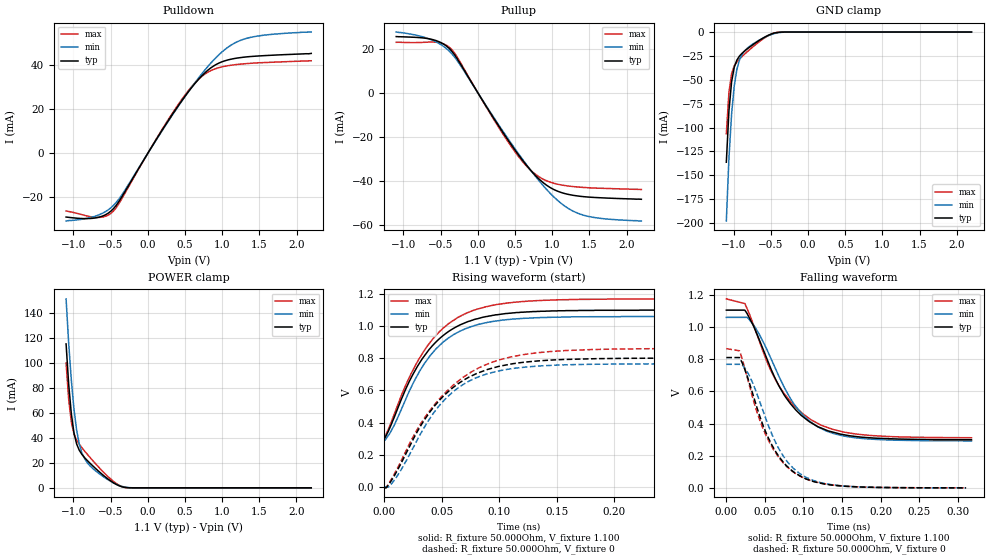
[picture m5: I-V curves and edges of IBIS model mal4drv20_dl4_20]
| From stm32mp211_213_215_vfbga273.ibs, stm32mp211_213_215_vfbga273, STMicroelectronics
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[Model] mal4drv20_dl4_20
Model_type   I/O
Polarity   Non-Inverting
Enable   Active-High
C_comp   1.837pF   1.837pF   1.849pF
C_comp_pullup   942.491fF   934.703fF   950.576fF
C_comp_pulldown 782.742fF   781.933fF   799.826fF
Vinh = 453.000mV
Vinl = 333.000mV
Vmeas = 393.000mV
Vref = 0.00V
Rref = 50Ohms
Cref = 0pF
[Model Spec]
Vinh   453.000mV   439.000mV   478.000mV
Vinl   333.000mV   319.000mV   358.000mV
Vmeas   393.000mV   379.000mV   418.000mV
Vref   0.00V   0.00V   0.00V
D_overshoot_ampl_h 0.3 NA   NA
D_overshoot_ampl_l 0.3 NA   NA
D_overshoot_area_l 100.000m NA   NA
D_overshoot_area_h 100.000m NA   NA
[Receiver Thresholds]
Vth = 393.000mV
Vth_min = 379.000mV
Vth_max = 418.000mV
Vinh_ac = 600.000mV
Vinh_dc = 600.000mV
Vinl_ac = -600.000mV
Vinl_dc = -600.000mV
Tslew_ac = 5.000ns
Threshold_sensitivity = 0.5
Reference_supply Pullup_ref
[Temperature Range]   25.000   125.000   -40.000
[Voltage Range]   1.100V   1.060V   1.170V
[GND Clamp Reference]   0.00V   0.00V   0.00V
[C Comp Corner]
| variable   typ   min   max
C_comp 1.849pF   1.837pF   1.837pF
C_comp_pullup 942.491fF   950.576fF   934.703fF
C_comp_pulldown 781.933fF   799.826fF   782.742fF
[Pulldown Reference]   0.00V   0.00V   0.00V
[POWER Clamp Reference]   1.100V   1.060V   1.170V
[Pullup Reference]   1.100V   1.060V   1.170V
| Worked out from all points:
|   slope of the pulldown table from 0 to 0.165 V, typ, clamps not added: 18.3 ohm
|   slope of the pullup table from 0 to 0.165 V, typ, clamps not added: 18.3 ohm
|   GND clamp passes 1 mA (typ) near -0.45 V on its own axis
|   POWER clamp passes 1 mA (typ) near -0.36 V on its own axis
|   rising waveform, R_fixture 50.000Ohm, V_fixture 1.100: 20-80 % time 40.7ps typ, 39.5ps min, 42.7ps max; typ from 0.296 V to 1.1 V
|   rising waveform, R_fixture 50.000Ohm, V_fixture 0: 20-80 % time 48.5ps typ, 45.1ps min, 54.6ps max; typ from -0.006 V to 0.802 V
|   falling waveform, R_fixture 50.000Ohm, V_fixture 1.100: 20-80 % time 54.3ps typ, 52.8ps min, 57.7ps max; typ from 1.1 V to 0.299 V
|   falling waveform, R_fixture 50.000Ohm, V_fixture 0: 20-80 % time 43.2ps typ, 43.3ps min, 43.7ps max; typ from 0.81 V to 0 V
[GND Clamp]
-1.099V   -136.3mA   -197.9mA   -106.5mA
-1.064V   -82.47mA   -132mA     -62.93mA
-1.028V   -52.05mA   -85.75mA   -43.61mA
-992.7mV  -36.88mA   -56.43mA   -35.5mA
-957.3mV  -29.36mA   -39.14mA   -31.26mA
-921.8mV  -25.1mA    -29.22mA   -28.2mA
-886.4mV  -22.16mA   -23.33mA   -25.51mA
-850.9mV  -19.73mA   -19.54mA   -22.95mA
-780mV    -15.43mA   -14.59mA   -18.04mA
-531.8mV  -3.288mA   -3.748mA   -3.604mA
-390mV    -251.1uA   -613.4uA   -163.8uA
2.198V    42.3nA     621.2nA    4.643nA
[Power Clamp]
-1.098V   115.5mA    151.6mA    100.1mA
-1.063V   83.06mA    116mA      70.82mA
-1.027V   59.24mA    86.19mA    52.7mA
-991.8mV  44.02mA    63.02mA    43.29mA
-956.4mV  35.26mA    46.38mA    38.3mA
-920.9mV  30.19mA    35.27mA    34.98mA
-885.5mV  26.87mA    28.15mA    32.19mA
-850mV    24.29mA    23.52mA    29.6mA
-672.7mV  13.97mA    12.28mA    17.45mA
-424.5mV  2.786mA    2.91mA     3.554mA
-282.7mV  160.9uA    380.1uA    143.1uA
2.199V    -14.13nA   -533.6nA   -2.884nA
[Pulldown]
-1.099V   -28.9mA    -30.7mA    -26.1mA
-673.6mV  -29.1mA    -28.13mA   -29.08mA
-567.3mV  -27.84mA   -26.4mA    -28.55mA
-460.9mV  -25.07mA   -23.59mA   -26.16mA
-319.1mV  -18.05mA   -17.33mA   -18.8mA
106.4mV   5.844mA    5.694mA    6.058mA
425.4mV   22.34mA    22.12mA    22.91mA
673.6mV   33.21mA    33.77mA    33.29mA
886.4mV   39.63mA    42.33mA    38.06mA
1.099V    42.53mA    48.61mA    39.85mA
1.312V    43.67mA    51.97mA    40.64mA
2.198V    45.3mA     55mA       41.97mA
[Pullup]
-1.098V   25.6mA     27.67mA    23mA
-637.3mV  24.46mA    24.31mA    23.1mA
-495.5mV  22.84mA    21.93mA    22.66mA
-389.1mV  20.32mA    19.12mA    20.9mA
-282.7mV  15.79mA    14.9mA     16.56mA
213.6mV   -11.6mA    -11.2mA    -12.1mA
532.7mV   -27.64mA   -27.1mA    -28.38mA
745.5mV   -36.64mA   -36.8mA    -36.33mA
958.2mV   -42.86mA   -45.26mA   -40.53mA
1.206V    -46.2mA    -52.45mA   -42.41mA
1.419V    -47.3mA    -55.72mA   -43.1mA
2.199V    -48.5mA    -58.4mA    -44.03mA
[Ramp]
R_load=50.000Ohm
dV/dt_r   480.930mV/45.500ps  460.349mV/43.500ps  516.120mV/50.000ps
dV/dt_f   480.930mV/49.500ps  460.349mV/49.000ps  516.120mV/51.500ps
[Rising waveform]
R_fixture=50.000Ohm
V_fixture=1.100
V_fixture_min=1.060
V_fixture_max=1.170
0s        296.5mV    285.5mV    301.3mV
9ps       434.7mV    385.1mV    453.9mV
19ps      610.6mV    547.3mV    634.8mV
26ps      711.2mV    655.1mV    739mV
35ps      814.6mV    766.6mV    848.7mV
51ps      939.9mV    899mV      985.3mV
72ps      1.026V     987.7mV    1.083V
98ps      1.071V     1.033V     1.135V
132ps     1.091V     1.052V     1.159V
294ps     1.1V       1.06V      1.17V
[Rising waveform]
R_fixture=50.000Ohm
V_fixture=0
0s        -5.912mV   -67.88uV   -3.484mV
4ps       12.81mV    -67.88uV   18.56mV
10ps      81.76mV    51.19mV    93.36mV
29ps      345.3mV    293.7mV    359.3mV
47ps      529.7mV    496.9mV    538.4mV
67ps      654.6mV    629.1mV    672.9mV
91ps      733.1mV    706.5mV    768.3mV
115ps     770mV      739.7mV    815.9mV
154ps     792.2mV    758.9mV    846.9mV
296ps     801.6mV    765.9mV    861.3mV
[Falling waveform]
R_fixture=50.000Ohm
V_fixture=1.100
V_fixture_min=1.060
V_fixture_max=1.170
0s        1.105V     1.06V      1.175V
24ps      1.105V     1.06V      1.146V
33ps      1.029V     1.028V     1.042V
52ps      808.4mV    866.2mV    793.4mV
68ps      635.4mV    695.6mV    637.1mV
88ps      495.5mV    519.9mV    510.6mV
110ps     404.8mV    407.6mV    422.8mV
129ps     359.9mV    354.7mV    378.8mV
166ps     320.4mV    311.9mV    336mV
318ps     299.2mV    292mV      311.5mV
[Falling waveform]
R_fixture=50.000Ohm
V_fixture=0
0s        810.1mV    768.2mV    865.5mV
17ps      810.1mV    768.2mV    852.3mV
24ps      736.1mV    745.2mV    743.3mV
39ps      509.9mV    593.8mV    481.3mV
51ps      348.2mV    433.2mV    330.7mV
70ps      183.4mV    226.9mV    176.2mV
88ps      96.67mV    117.1mV    94.18mV
112ps     40.68mV    47.39mV    41.68mV
146ps     12.88mV    13.8mV     13.76mV
311ps     112.7uV    145.4uV    117.1uV
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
